(* Logix 5000 AddOnInstructionDefinition export; software revision 16.04 *)

ADD_ON_INSTRUCTION AMCI_ANG1E_Enable_Driver   (* revision 1.1, vendor AMCI *)
// Revision note:
// Version 1.1 added the slot_axis number and the input parameters can now be tags or discrete values.
VAR_INPUT
   slot_axis_number : INT; {required}
END_VAR
VAR_IN_OUT
   AMCI_ANG1E_output_data : INT[10]; {required}
END_VAR
VAR
   command_data_block : INT[10];
        [0]   // Command Bits MSW
        [1]   // Command Bits LSW
        [2]   // Upper Target Position
        [3]   // Lower Target Position
        [4]   // Upper Programmed Speed
        [5]   // Lower Programmed Speed
   index : INT;
END_VAR

ROUTINE Logic   (* ladder *)
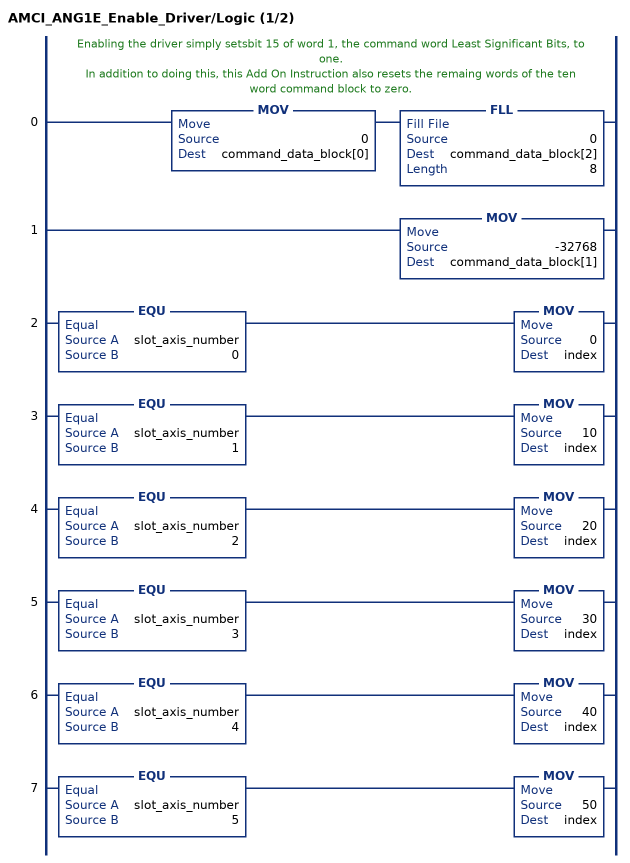
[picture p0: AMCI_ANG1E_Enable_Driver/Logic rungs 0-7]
   // Enabling the driver simply setsbit 15 of word 1, the command word Least Significant Bits, to one.
   // In addition to doing this, this Add On Instruction also resets the remaing words of the ten word command block to zero.
   0: MOV(0,command_data_block[0])FLL(0,command_data_block[2],8);
   1: MOV(-32768,command_data_block[1]);
   2: EQU(slot_axis_number,0)MOV(0,index);
   3: EQU(slot_axis_number,1)MOV(10,index);
   4: EQU(slot_axis_number,2)MOV(20,index);
   5: EQU(slot_axis_number,3)MOV(30,index);
   6: EQU(slot_axis_number,4)MOV(40,index);
   7: EQU(slot_axis_number,5)MOV(50,index);
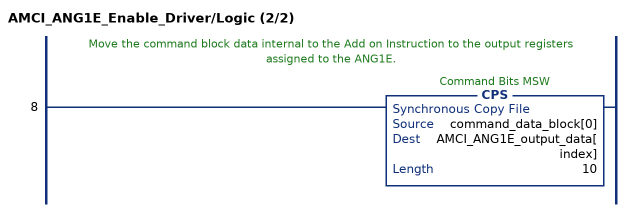
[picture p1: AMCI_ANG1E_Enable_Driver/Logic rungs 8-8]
   // Move the command block data internal to the Add on Instruction to the output registers assigned to the ANG1E.
   8: CPS(command_data_block[0],AMCI_ANG1E_output_data[index],10);
END_ROUTINE
END_ADD_ON_INSTRUCTION
